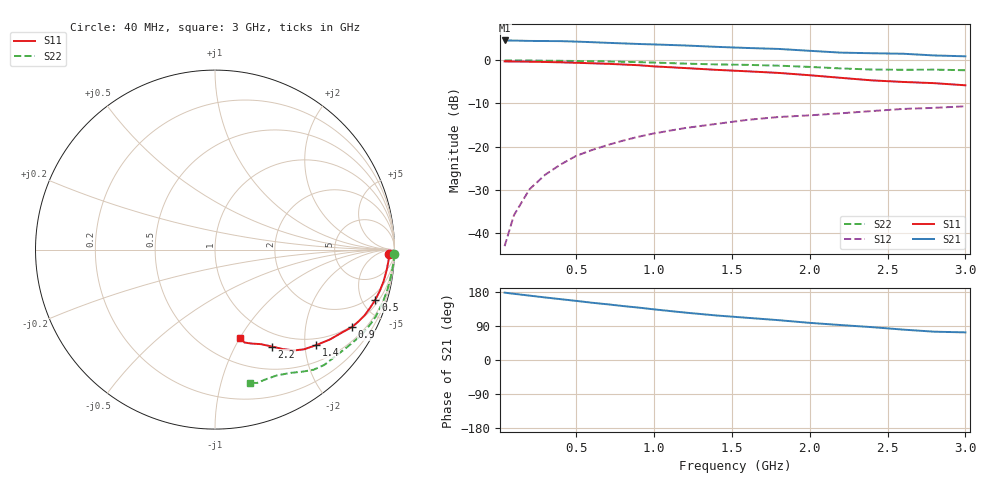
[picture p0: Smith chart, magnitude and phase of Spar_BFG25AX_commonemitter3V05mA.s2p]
! Filename:  BFG25AXH.S2P  Version:  2.0
! NXP part #: BFG25A/X  Date: May 1990
! Bias condition: Vce=3V, Ic=0.5mA
#  MHz  S  MA  R  50
! Freq  S11  S21  S12  S22  !GUM [dB]
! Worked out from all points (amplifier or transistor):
!   21 points, 40 MHz to 3 GHz, reference 50 ohm
!   highest |S21| = 4.6 dB at 40 MHz (marker M1)
!   |S21| within 3 dB of that: start of sweep to 2.461 GHz
!   unconditionally stable (mu >= 1): nowhere
!   at 300 MHz: K = 0.09, MSG = 15.5 dB, |S12| = -26.6 dB
!   at 1 GHz: K = 0.26, MSG = 10.3 dB, |S12| = -17.0 dB
!   at 3 GHz: K = 0.68, MSG = 5.8 dB, |S12| = -10.7 dB
!   lowest NFmin = 1.50 dB at 500 MHz
!   S11 on the Smith chart (normalised r, x): 40 MHz: 42, -31; 500 MHz: 1.40, -6.27; 900 MHz: 0.95, -3.56; 1.4 GHz: 0.84, -2.24; 2.2 GHz: 0.80, -1.42; 3 GHz: 0.75, -1.01
40  0.97 -1.3  1.698 177.8  0.007 86.7  0.999 -1.3
100  0.969 -3.5  1.694 174.7  0.016 87.5  0.998 -3.4
200  0.963 -6.9  1.677 169.9  0.032 84.4  0.994 -6.7
300  0.956 -10.6  1.672 165.1  0.047 81.8  0.99 -10.1
400  0.947 -14.0  1.668 160.5  0.062 79.3  0.986 -13.3
500  0.936 -17.3  1.647 156.0  0.078 77.3  0.981 -16.6
600  0.923 -20.6  1.622 151.2  0.091 75.2  0.975 -19.7
700  0.911 -23.6  1.594 147.0  0.104 73.3  0.97 -22.7
800  0.894 -26.6  1.57 142.4  0.117 71.6  0.961 -25.5
900  0.877 -29.5  1.546 138.3  0.13 69.5  0.951 -28.2
1000  0.85 -32.5  1.527 133.6  0.142 67.4  0.941 -31.0
1200  0.813 -38.0  1.485 125.1  0.164 62.8  0.915 -36.4
1400  0.775 -43.4  1.432 117.5  0.183 59.6  0.896 -41.6
1600  0.745 -48.2  1.389 111.3  0.204 57.1  0.885 -46.6
1800  0.714 -51.9  1.354 105.1  0.22 53.8  0.866 -50.6
2000  0.671 -55.7  1.288 98.0  0.23 50.9  0.838 -54.2
2200  0.626 -59.6  1.227 92.2  0.243 48.3  0.805 -58.6
2400  0.585 -64.2  1.207 86.7  0.258 44.8  0.781 -63.9
2600  0.561 -68.9  1.191 80.2  0.273 41.4  0.776 -68.9
2800  0.543 -72.4  1.138 74.7  0.281 40.0  0.779 -72.5
3000  0.513 -74.0  1.112 72.9  0.293 39.9  0.767 -75.3
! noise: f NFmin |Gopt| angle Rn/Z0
500  1.5  0.88  4  3
1000  1.6  0.8  13  3.2
2000  1.8  0.79  37  2.2
